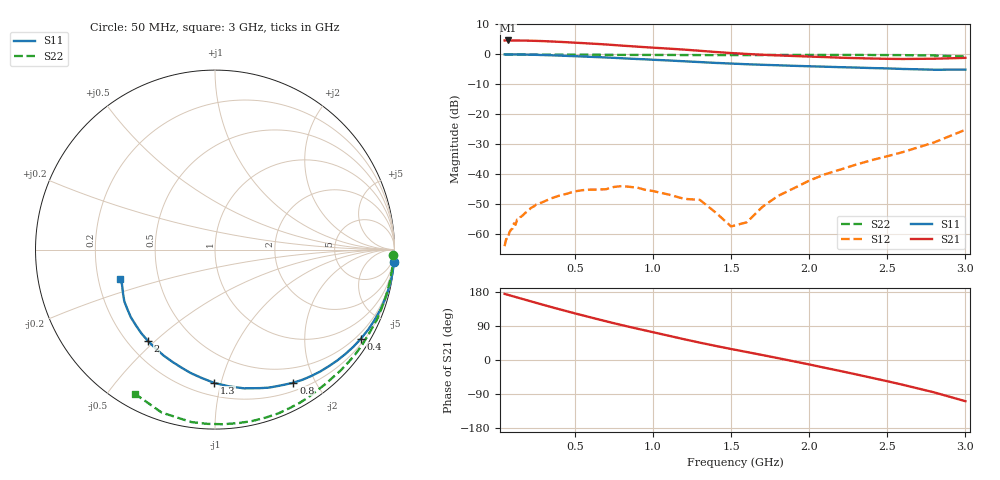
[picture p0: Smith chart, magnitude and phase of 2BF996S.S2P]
! BF996S Si-Dual Gate MOS-FET in SOT143 package
! V ds = 15V  I d = 10mA  V g2= 4V
# GHZ S MA R 50
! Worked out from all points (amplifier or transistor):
!   50 points, 50 MHz to 3 GHz, reference 50 ohm
!   highest |S21| = 4.6 dB at 70 MHz (marker M1)
!   |S21| within 3 dB of that: start of sweep to 1.182 GHz
!   unconditionally stable (mu >= 1): 715.7 MHz to 2.066 GHz
!   at 130 MHz: K = 0.15, MSG = 29.9 dB, |S12| = -55.2 dB
!   at 700 MHz: K = 0.98, MSG = 24.2 dB, |S12| = -45.1 dB
!   at 3 GHz: K = 0.64, MSG = 12.0 dB, |S12| = -25.2 dB
!   S11 on the Smith chart (normalised r, x): 50 MHz: 1, -29; 400 MHz: 0.33, -3.53; 800 MHz: 0.30, -1.71; 1.3 GHz: 0.29, -0.95; 2 GHz: 0.28, -0.48; 3 GHz: 0.29, -0.14
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0.05  0.9984 -4.0  1.703 174.4  0.000624 92.3  0.9936 -1.7
0.06  0.9985 -4.8  1.705 173.3  0.000822 89.3  0.9936 -2.1
0.07  0.9982 -5.6  1.705 172.1  0.00082 86.0  0.9935 -2.4
0.08  0.9979 -6.4  1.704 170.9  0.001055 82.5  0.9933 -2.7
0.11  0.9962 -8.8  1.703 167.5  0.001497 83.4  0.9935 -3.8
0.12  0.9954 -9.6  1.704 166.3  0.001421 83.5  0.9929 -4.1
0.13  0.9947 -10.4  1.702 165.1  0.001733 82.7  0.9931 -4.5
0.25  0.9807 -19.9  1.678 151.1  0.003072 75.4  0.9914 -8.5
0.4  0.9527 -31.4  1.617 134.0  0.004357 65.4  0.9873 -13.6
0.55  0.9195 -42.2  1.541 117.8  0.005382 57.5  0.9841 -18.6
0.7  0.8856 -52.6  1.461 102.2  0.005591 55.3  0.9826 -23.6
0.8  0.8604 -59.5  1.399 92.2  0.006292 50.3  0.9783 -26.8
1.1  0.7895 -78.2  1.246 64.1  0.004545 42.0  0.9754 -36.7
1.3  0.7424 -90.4  1.146 45.8  0.003701 47.1  0.9714 -43.9
1.5  0.7011 -101.1  1.051 29.1  0.001333 85.5  0.9691 -50.8
1.6  0.6835 -105.9  1.015 21.1  0.001563 135.0  0.9698 -54.2
1.8  0.6562 -115.8  0.9609 4.9  0.004306 167.4  0.9757 -61.2
2  0.6317 -126.2  0.9179 -11.7  0.00776 174.9  0.9786 -68.9
2.1  0.6213 -131.3  0.8993 -20.5  0.009881 176.7  0.9776 -73.1
2.6  0.5697 -153.9  0.8359 -65.4  0.0233 -176.6  0.97 -97.8
2.8  0.5533 -159.5  0.845 -85.4  0.03376 -171.1  0.9553 -108.1
3  0.5547 -163.1  0.8721 -108.7  0.0549 -170.7  0.9189 -119.1
